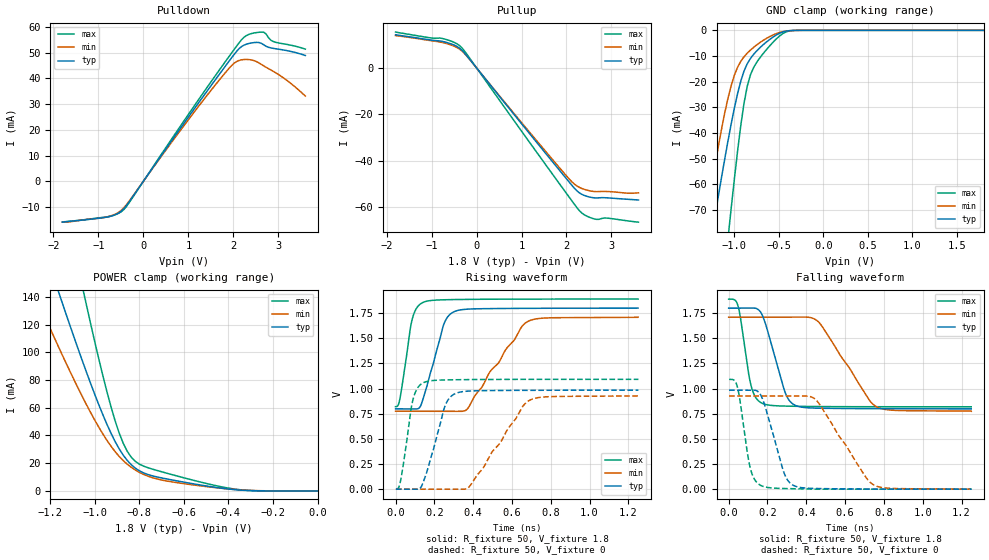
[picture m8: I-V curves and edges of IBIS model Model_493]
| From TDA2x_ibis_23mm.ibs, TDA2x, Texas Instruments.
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| Model based on original model for DDR_DIFFIOPB_H
|   Sub model SR000_DRV40_1P8
[model]   Model_493
|[Description]  [1.8V-I/O-X-X]
|   , ,
|[Input Load]
|[Output Drive]
|Voltage   1.8V
|Mode   I/O
Model_type   I/O
Polarity   Non-Inverting
Enable   Active-Low
Vinl =  0.775
Vinh =  1.025
Cref =  15.0000pF
Rref =  100.0000M
Vref =  0V
Vmeas =  0.9
C_comp   2p   2p   2p
[Model Spec]
Vinl   0.78   0.735   0.825
Vinh   1.02   0.975   1.065
[Receiver Thresholds]
Tslew_ac = 0.5n
Vth= 0.9
Vth_max= 0.945
Vth_min= 0.81
Vinh_ac= 0.2
Vinh_dc= 0.125
Vinl_ac= -0.2
Vinl_dc= -0.125
[Temperature Range]   25   125   -40
[Voltage Range]   1.8   1.71   1.89
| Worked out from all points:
|   slope of the pulldown table from 0 to 0.27 V, typ, clamps not added: 39.7 ohm
|   slope of the pullup table from 0 to 0.27 V, typ, clamps not added: 41.4 ohm
|   GND clamp passes 1 mA (typ) near -0.48 V on its own axis
|   POWER clamp passes 1 mA (typ) near -0.38 V on its own axis
|   rising waveform, R_fixture 50, V_fixture 1.8: 20-80 % time 83.9ps typ, 201ps min, 49.9ps max; typ from 0.799 V to 1.8 V
|   rising waveform, R_fixture 50, V_fixture 0: 20-80 % time 82.9ps typ, 191ps min, 49.8ps max; typ from 0 V to 0.984 V
|   falling waveform, R_fixture 50, V_fixture 1.8: 20-80 % time 87.8ps typ, 186ps min, 51.9ps max; typ from 1.8 V to 0.799 V
|   falling waveform, R_fixture 50, V_fixture 0: 20-80 % time 85.8ps typ, 182ps min, 51.3ps max; typ from 0.984 V to 0 V
[POWER_clamp]
-1.8V     464.6mA    344.4mA    740.8mA
-1.273V   197mA      143.3mA    314.4mA
-1.164V   144mA      104.2mA    229mA
-1.145V   135.3mA    97.86mA    215mA
-1.055V   93.25mA    67.59mA    146.5mA
-1.036V   85.18mA    61.89mA    133.3mA
-909.1mV  35.72mA    28.41mA    50.73mA
-872.7mV  25.87mA    21.94mA    34.5mA
-818.2mV  16.45mA    15.08mA    21.33mA
-690.9mV  9.084mA    7.592mA    13.42mA
-400mV    1.38mA     1.43mA     2.039mA
0V        227.3nA    761nA      1.176uA
[Pulldown]
-1.8V     -15.9mA    -15.92mA   -15.81mA
-818.2mV  -13.96mA   -13.89mA   -13.92mA
-600mV    -12.8mA    -12.58mA   -12.84mA
-436.4mV  -10.71mA   -10.33mA   -11.03mA
1.255V    31.16mA    29.78mA    32.45mA
1.855V    45.52mA    42.91mA    47.32mA
2.073V    50.52mA    46.55mA    52.56mA
2.291V    53.3mA     47.36mA    56.66mA
2.618V    53.66mA    45.48mA    58mA
2.727V    52.47mA    44.31mA    57.26mA
2.891V    51.66mA    42.7mA     54.29mA
3.6V      48.88mA    33.12mA    51.37mA
[Pullup]
-1.8V     14.28mA    13.9mA     15.42mA
-1.036V   12.05mA    11.79mA    12.97mA
-763.6mV  11.43mA    10.95mA    12.69mA
-381.8mV  8.556mA    8.124mA    9.674mA
-218.2mV  5.258mA    5.122mA    5.967mA
2.018V    -48.25mA   -46.99mA   -54.63mA
2.182V    -52.02mA   -50.21mA   -58.98mA
2.291V    -53.95mA   -51.57mA   -61.66mA
2.455V    -55.39mA   -52.71mA   -63.95mA
2.673V    -56.09mA   -53.37mA   -65.34mA
2.891V    -56.02mA   -53.3mA    -64.76mA
3.6V      -56.97mA   -53.87mA   -66.53mA
[GND_clamp]
-1.8V     -200.8mA   -187.9mA   -345.9mA
-1.327V   -95.75mA   -76.22mA   -171.1mA
-1.255V   -80.19mA   -60.47mA   -144.9mA
-1.218V   -72.53mA   -52.92mA   -131.9mA
-1.073V   -43.32mA   -26.59mA   -81.54mA
-1.036V   -36.61mA   -21.6mA    -69.55mA
-963.6mV  -24.61mA   -14.37mA   -47.01mA
-854.5mV  -12.98mA   -8.864mA   -21.66mA
-781.8mV  -9.263mA   -6.573mA   -14.36mA
-672.7mV  -5.498mA   -3.827mA   -8.897mA
-345.5mV  -48.81uA   -73.08uA   -79.37uA
1.8V      227.3nA    3.986uA    988nA
[Ramp]
dV/dt_f 0.60152695/87.856657p 0.56188703/0.18590935n 0.64274256/51.891391p
dV/dt_r 0.59179499/83.073453p 0.55709331/0.19106712n 0.65655366/49.898971p
R_load = 50
[Rising Waveform]
R_fixture = 50
V_fixture = 1.8
V_fixture_min = 1.71
V_fixture_max = 1.89
0s        798.6mV    774.9mV    820.1mV
22.93ps   798.1mV    774.8mV    902.7mV
86.93ps   797.8mV    774.8mV    1.697V
122.5ps   808.4mV    774.8mV    1.833V
142.8ps   902.9mV    774.8mV    1.858V
248ps     1.635V     774.6mV    1.883V
304.9ps   1.767V     774.1mV    1.885V
371.5ps   1.79V      800.7mV    1.887V
682.4ps   1.798V     1.668V     1.89V
1.25ns    1.8V       1.71V      1.89V
[Rising Waveform]
R_fixture = 50
V_fixture = 0
V_fixture_min = 0
V_fixture_max = 0
1.951ps   0V         0V         0V
27.09ps   0V         0V         94.7mV
90.25ps   0V         0V         894.2mV
125.6ps   7.783mV    0V         1.035V
145.2ps   82.49mV    0V         1.06V
253.2ps   817.8mV    0V         1.086V
311.1ps   953.1mV    0V         1.088V
382.6ps   975.8mV    30.5mV     1.09V
692.2ps   982.8mV    885.1mV    1.092V
1.252ns   984.5mV    926.8mV    1.092V
[Falling Waveform]
R_fixture = 50
V_fixture = 1.8
V_fixture_min = 1.71
V_fixture_max = 1.89
0s        1.8V       1.71V      1.89V
46.56ps   1.8V       1.71V      1.833V
115.5ps   1.8V       1.71V      1.029V
139.3ps   1.799V     1.71V      911.9mV
173.9ps   1.728V     1.71V      852.8mV
290.4ps   966.1mV    1.71V      826.1mV
344.5ps   832.6mV    1.71V      824mV
467ps     805mV      1.655V     821.4mV
763.5ps   800.3mV    818.1mV    819.6mV
1.25ns    798.6mV    774.9mV    819.3mV
[Falling Waveform]
R_fixture = 50
V_fixture = 0
V_fixture_min = 0
V_fixture_max = 0
1.951ps   984.5mV    926.8mV    1.092V
42.52ps   984.7mV    926.9mV    1.033V
110ps     984.3mV    926.9mV    219.7mV
133.8ps   984.9mV    926.9mV    95.32mV
168.3ps   924.8mV    926.8mV    34.21mV
284.8ps   165.1mV    926.8mV    6.377mV
338.4ps   33.29mV    926.5mV    4.066mV
455.5ps   6.319mV    876.8mV    0V
749.5ps   0V         40.08mV    0V
1.252ns   0V         0V         0V
